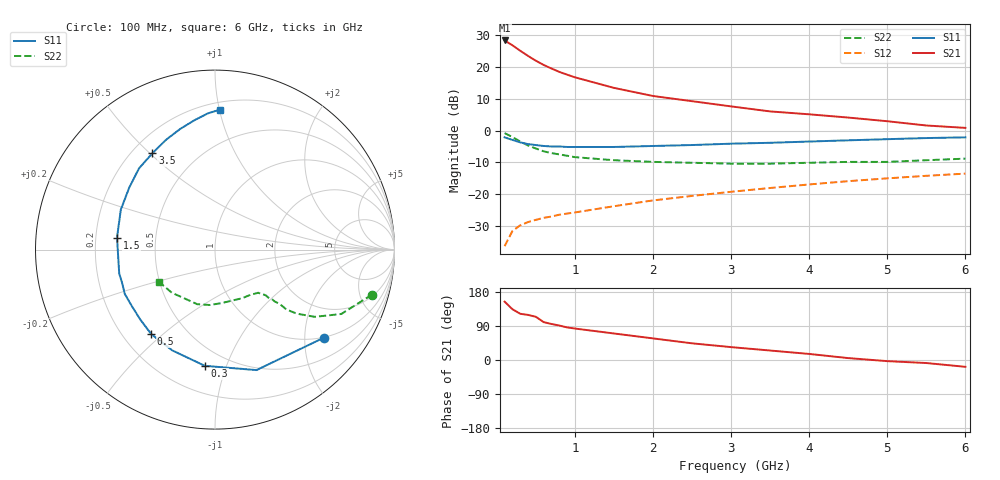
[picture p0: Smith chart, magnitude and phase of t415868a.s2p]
!AT-41586
!S-PARAMETERS at Vce=8V Ic=10mA. LAST UPDATED 08-03-92
# ghz s ma r 50
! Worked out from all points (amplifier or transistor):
!   20 points, 100 MHz to 6 GHz, reference 50 ohm
!   highest |S21| = 28.4 dB at 100 MHz (marker M1)
!   |S21| within 3 dB of that: start of sweep to 285.8 MHz
!   unconditionally stable (mu >= 1): 1.574 GHz to 3.714 GHz
!   at 400 MHz: K = 0.41, MSG = 26.2 dB, |S12| = -28.9 dB
!   at 1.5 GHz: K = 0.99, MSG = 18.7 dB, |S12| = -23.9 dB
!   at 6 GHz: K = 0.78, MSG = 7.2 dB, |S12| = -13.6 dB
!   lowest NFmin = 1.30 dB at 100 MHz
!   S11 on the Smith chart (normalised r, x): 100 MHz: 0.99, -2.48; 300 MHz: 0.38, -0.84; 500 MHz: 0.32, -0.46; 1.5 GHz: 0.29, +0.06; 3.5 GHz: 0.28, +0.51; 6 GHz: 0.25, +1.00
0.1  0.78 -39.0  26.3 154.0  0.015 71.0  0.91 -16.0
0.2  0.71 -71.0  22.1 134.0  0.026 59.0  0.79 -27.0
0.3  0.65 -95.0  18.1 122.0  0.032 50.0  0.67 -34.0
0.4  0.61 -113.0  15 119.0  0.036 44.0  0.58 -38.0
0.5  0.59 -127.0  12.6 114.0  0.039 43.0  0.52 -40.0
0.6  0.57 -137.0  10.8 100.0  0.042 43.0  0.47 -40.0
0.7  0.56 -146.0  9.5 95.0  0.044 43.0  0.44 -41.0
0.8  0.56 -154.0  8.4 91.0  0.047 43.0  0.42 -41.0
0.9  0.55 -160.0  7.6 86.0  0.049 44.0  0.4 -42.0
1  0.55 -166.0  6.9 83.0  0.051 47.0  0.38 -42.0
1.5  0.55 173.0  4.7 70.0  0.064 49.0  0.34 -45.0
2  0.57 157.0  3.5 57.0  0.079 49.0  0.32 -52.0
2.5  0.59 144.0  2.9 44.0  0.093 48.0  0.31 -61.0
3  0.62 133.0  2.4 34.0  0.108 47.0  0.3 -71.0
3.5  0.64 123.0  2 25.0  0.124 45.0  0.3 -83.0
4  0.67 114.0  1.8 16.0  0.141 42.0  0.31 -95.0
4.5  0.7 106.0  1.6 5.0  0.159 39.0  0.32 -108.0
5  0.73 99.0  1.4 -3.0  0.176 35.0  0.32 -121.0
5.5  0.76 93.0  1.2 -8.0  0.193 31.0  0.34 -135.0
6  0.78 88.0  1.1 -18.0  0.209 31.0  0.36 -150.0
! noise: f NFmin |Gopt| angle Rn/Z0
0.1  1.3  0.12  3  0.17
0.5  1.3  0.1  16  0.17
1  1.4  0.04  43  0.16
2  1.7  0.12  -145  0.16
